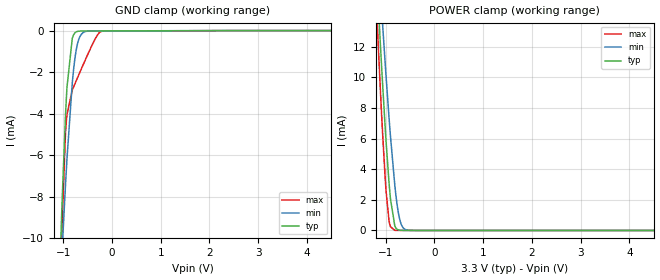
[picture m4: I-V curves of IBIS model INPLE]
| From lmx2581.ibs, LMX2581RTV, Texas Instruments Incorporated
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[Model]   INPLE
Model_type   Input
Vinl = .4
Vinh = 1.4
|   typ   min   max
|   (nom PVT)   (slow PVT)   (fast PVT)
C_comp   0.097p   0.055p   0.172p
[Voltage Range]   3.3   3   3.6
[Temperature Range]   27   125   -40
[Power Clamp Reference]   3.3   3   3.6
[GND Clamp Reference]   0   0   0
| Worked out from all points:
|   GND clamp passes 1 mA (typ) near -0.84 V on its own axis
|   POWER clamp passes 1 mA (typ) near -0.85 V on its own axis
[GND Clamp]
|   Voltage   I(typ)   I(min)   I(max)
-3.3V     -246.7mA   -151.3mA   -472.5mA
-1.063V   -11mA      -12.48mA   -13.39mA
-1.043V   -9.539mA   -11.5mA    -11.16mA
-1.033V   -8.836mA   -11.02mA   -10.16mA
-1.023V   -8.153mA   -10.55mA   -9.224mA
-953.7mV  -4.049mA   -7.405mA   -4.889mA
-924mV    -2.732mA   -6.176mA   -4.04mA
-815.1mV  -371.5uA   -2.519mA   -2.869mA
-726mV    -52.96uA   -830uA     -2.372mA
-597.3mV  -21.95uA   -105.1uA   -1.676mA
-211.2mV  -18.93uA   -16.52uA   -33.92uA
6.6V      0A         0A         0A
[POWER Clamp]
|   Voltage   I(typ)   I(min)   I(max)
-3.3V     164.1mA    142.7mA    184.6mA
-1.27V    21.96mA    24.02mA    20.36mA
-1.162V   15.17mA    18.3mA     12.58mA
-1.112V   12.23mA    15.78mA    9.26mA
-1.073V   9.965mA    13.81mA    6.77mA
-993.3mV  5.787mA    10.03mA    2.551mA
-924mV    2.769mA    6.983mA    476uA
-815.1mV  302.8uA    2.97mA     12.8uA
-755.7mV  56.91uA    1.434mA    5.354uA
-696.3mV  12.57uA    526.6uA    4.188uA
-537.9mV  2.868uA    18.98uA    2.42uA
6.6V      0A         0A         0A
